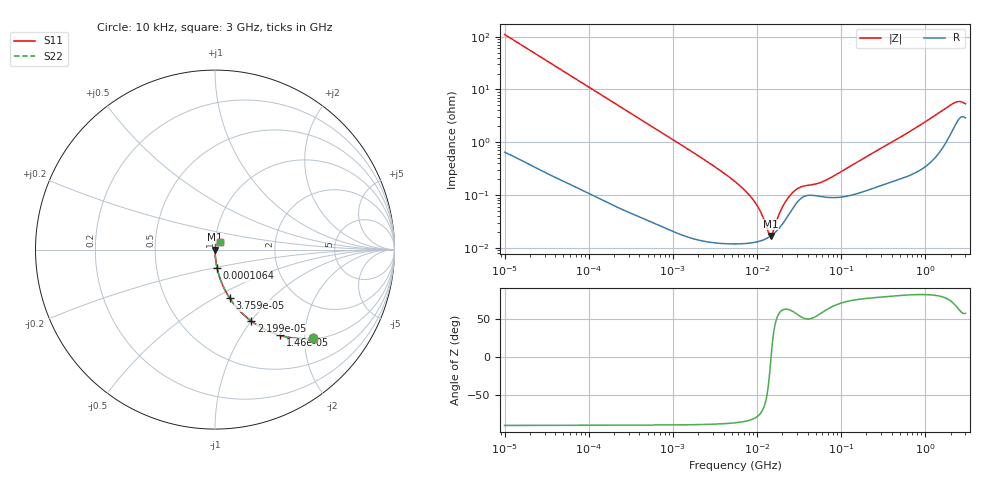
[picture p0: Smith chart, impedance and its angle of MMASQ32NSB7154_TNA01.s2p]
! MMASQ32NSB7154_TNA01  S-PARAMETER MODEL  ( Standard Model )
! Model Generated by TAIYO YUDEN Corporation (http://www.ty-top.com)
! Version 1.0
! TAIYO YUDEN Control No. 220601
! Copyright(c) 2013 TAIYO YUDEN CO.,LTD. All Rights Reserved.
! Product Description (link to TY-COMPAS)
! https://ds.yuden.co.jp/TYCOMPAS/or/detail?pn=MMASQ32NSB7154KTNA01&u=M
! Products Name : Multilayer Ceramic Capacitors
! Characteristics :
!  Capacitance : 0.15 [uF] , Rated Voltage : 250 [V] , TCC : X7R
!  Case Size : 3.2 x 2.5 / 0.126 x 0.098 [mm/inch] , Thickness : 1.9 / 0.075 [mm/inch]
!  (Conditions: Temperature = 25 [degC] , DC Bias Voltage = 0 [V])
! External Node Assignments :
!  1  o---| |---o  2
! GND o---------o GND
! Frequency Range : 10kHz  -  3GHz  [ 401 STEP ]
# MHZ S RI R 50
! Freq[MHz].  S11 Real  S11 Imag  S21 Real  S21 Imag  S12 Real  S12 Imag  S22 Real  S22 Imag
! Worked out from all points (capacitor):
!   401 points, 10 kHz to 3 GHz, reference 50 ohm
!   read as one part in series: C = 145 nF near 10.65 kHz
!   lowest |Z| = 16.9 mohm at 14.56 MHz (marker M1)
!   series resonance near 14.7 MHz, so ESL is about 810 pH
!   S11 on the Smith chart (normalised r, x): 10 kHz: 1.01, -2.20; 14.6 kHz: 1.01, -1.51; 22 kHz: 1.01, -1.00; 37.59 kHz: 1.00, -0.59; 106.4 kHz: 1.00, -0.21; 3 GHz: 1.06, +0.09
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0.01  0.547 -0.4948  0.453 0.4948  0.453 0.4948  0.547 -0.4948
0.014599  0.3634 -0.4778  0.6366 0.4778  0.6366 0.4778  0.3634 -0.4778
0.021995  0.2026 -0.3985  0.7974 0.3985  0.7974 0.3985  0.2026 -0.3985
0.037592  0.0813 -0.2695  0.9187 0.2695  0.9187 0.2695  0.0813 -0.2695
0.082683  0.0189 -0.1315  0.9811 0.1315  0.9811 0.1315  0.0189 -0.1315
0.106405  0.0118 -0.1031  0.9882 0.1031  0.9882 0.1031  0.0118 -0.1031
0.683653  0.000538 -0.0164  0.9995 0.0164  0.9995 0.0164  0.000538 -0.0164
5.477226  0.000122 -0.0018  0.9999 0.0018  0.9999 0.0018  0.000122 -0.0018
9.6612  0.000129 -0.000684  0.9999 0.000684  0.9999 0.000684  0.000129 -0.000684
11.31085  0.000138 -0.000423  0.9999 0.000423  0.9999 0.000423  0.000138 -0.000423
13.66633  0.000158 -0.000117  0.9998 0.000117  0.9998 0.000117  0.000158 -0.000117
14.55585  0.000168 -1.54e-05  0.9998 1.54e-05  0.9998 1.54e-05  0.000168 -1.54e-05
15.50326  0.000181 8.77e-05  0.9998 -8.77e-05  0.9998 -8.77e-05  0.000181 8.77e-05
19.95104  0.00028 0.000513  0.9997 -0.000513  0.9997 -0.000513  0.00028 0.000513
24.87798  0.000477 0.000877  0.9995 -0.000877  0.9995 -0.000877  0.000477 0.000877
32.0153  0.00082 0.00112  0.9992 -0.00112  0.9992 -0.00112  0.00082 0.00112
45.28751  0.000992 0.00122  0.999 -0.00122  0.999 -0.00122  0.000992 0.00122
72.67256  0.000903 0.00187  0.9991 -0.00187  0.9991 -0.00187  0.000903 0.00187
374.4521  0.0018 0.00927  0.9982 -0.00927  0.9982 -0.00927  0.0018 0.00927
2120.803  0.0194 0.0492  0.9806 -0.0492  0.9806 -0.0492  0.0194 0.0492
2482.93  0.0286 0.0499  0.9714 -0.0499  0.9714 -0.0499  0.0286 0.0499
3000  0.03 0.0425  0.97 -0.0425  0.97 -0.0425  0.03 0.0425
